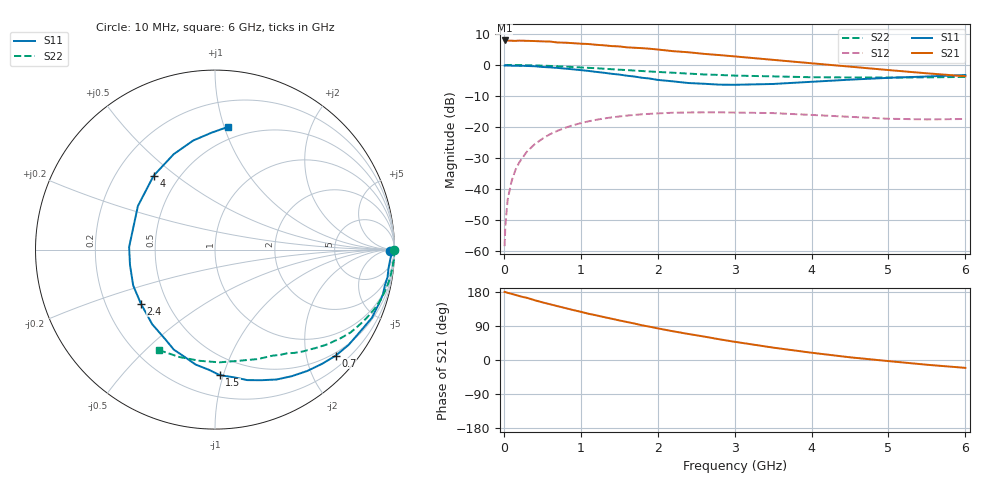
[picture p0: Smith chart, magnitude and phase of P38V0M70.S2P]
! SIEMENS Small Signal Semiconductors
! BFP181
! Si NPN RF Bipolar Junction Transistor in SOT143
! VCE = 8 V  IC = 0.7 mA
! Common Emitter S-Parameters:  March  1996
# GHz  S  MA  R  50
!  f  S11  S21  S12  S22
! GHz  MAG  ANG  MAG  ANG  MAG  ANG  MAG  ANG
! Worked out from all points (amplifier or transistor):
!   36 points, 10 MHz to 6 GHz, reference 50 ohm
!   highest |S21| = 7.9 dB at 10 MHz (marker M1)
!   |S21| within 3 dB of that: start of sweep to 2.03 GHz
!   unconditionally stable (mu >= 1): 3.609 GHz to end of sweep
!   at 250 MHz: K = 0.08, MSG = 18.7 dB, |S12| = -29.7 dB
!   at 1.4 GHz: K = 0.44, MSG = 11.5 dB, |S12| = -16.9 dB
!   at 6 GHz: K = 1.36, MAG = 3.3 dB, |S12| = -17.4 dB
!   S11 on the Smith chart (normalised r, x): 10 MHz: 70, -30; 700 MHz: 0.44, -2.59; 1.5 GHz: 0.35, -0.97; 2.4 GHz: 0.35, -0.29; 4 GHz: 0.36, +0.42; 6 GHz: 0.40, +1.03
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0.01  0.9762 -0.6  2.481 179.6  0.0012 90.6  0.9986 -0.2
0.02  0.9861 -1.5  2.475 179.3  0.0026 87.8  0.9909 -0.5
0.05  0.9786 -2.9  2.467 177.2  0.0068 92.5  0.9984 -1.5
0.1  0.9725 -6.1  2.457 174.6  0.0133 83.9  0.9999 -2.9
0.15  0.9734 -9.1  2.443 171.8  0.0202 83.1  0.9951 -4.3
0.3  0.9626 -18.0  2.445 164.1  0.0401 77.6  0.9886 -8.6
0.4  0.9531 -23.5  2.427 157.8  0.0526 73.9  0.9825 -11.4
0.6  0.9144 -35.5  2.384 147.1  0.0765 65.4  0.9643 -16.9
0.7  0.8952 -41.3  2.299 142.0  0.0871 61.5  0.952 -19.6
0.9  0.8496 -52.7  2.243 131.9  0.1071 54.0  0.9257 -24.4
1.1  0.8011 -64.6  2.175 122.1  0.1234 47.1  0.8984 -29.1
1.5  0.7001 -87.8  1.989 104.5  0.1476 34.8  0.8378 -37.4
1.9  0.6027 -112.4  1.823 87.7  0.163 24.6  0.7834 -44.5
2.2  0.5434 -130.1  1.667 75.8  0.1698 17.9  0.7489 -49.3
2.4  0.5111 -143.9  1.601 68.7  0.1713 13.6  0.7255 -52.5
2.8  0.4813 -169.7  1.443 54.7  0.1723 6.7  0.6898 -58.3
3  0.4787 178.3  1.373 48.1  0.1709 3.2  0.6732 -61.3
3.5  0.4935 150.5  1.208 32.7  0.1674 -3.3  0.6544 -68.8
4  0.5352 129.7  1.064 19.2  0.1565 -7.7  0.6335 -77.8
4.5  0.5793 113.4  0.939 7.1  0.1458 -10.9  0.6287 -87.7
5.5  0.6512 91.8  0.733 -12.5  0.1325 -7.9  0.6306 -108.4
6  0.6884 83.8  0.657 -20.8  0.1346 -5.3  0.6412 -119.3
